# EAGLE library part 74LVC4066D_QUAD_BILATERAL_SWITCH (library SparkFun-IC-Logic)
Nexperia Quad Bilateral Switch The 74LVC4066 is a high-speed Si-gate CMOS device. The 74LVC4066 provides four single pole, single-throw analog switch functions. Each switch has two input/output terminals (nY and nZ) and an active HIGH enable input (nE). When nE is LOW, the analog switch is turned off. Schmitt-trigger action at the enable inputs makes the circuit tolerant of slower input rise and fall times across the entire VCC range from 1.65 V to 5.5 V. Datasheet
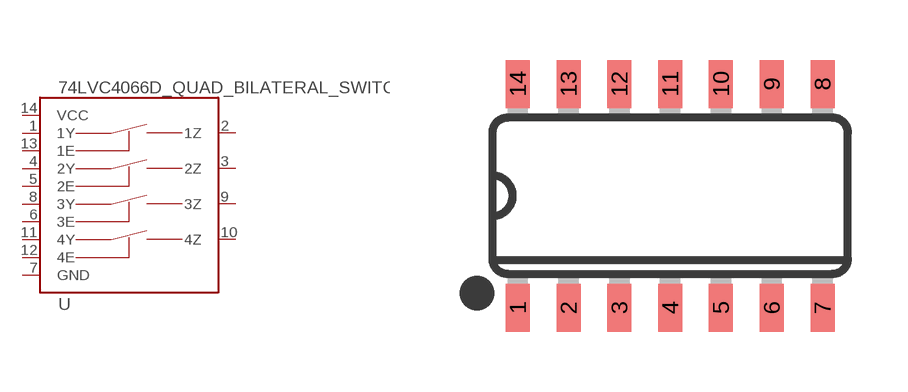
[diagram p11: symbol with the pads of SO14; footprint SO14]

Designator prefix U

## 74LVC4066D_QUAD_BILATERAL_SWITCH (PROD_ID: IC-13944)  [SO14]
1  1Y
2  1Z
3  2Z
4  2Y
5  2E
6  3E
7  GND
8  3Y
9  3Z
10  4Z
11  4Y
12  4E
13  1E
14  VCC

## Footprint SO14 (pad centres in mm)
smd 0.6 x 1.2: 1 -3.175,-2.8; 2 -1.905,-2.8; 3 -0.635,-2.8; 4 0.635,-2.8; 5 1.905,-2.8; 6 3.175,-2.8; 7 4.445,-2.8; 8 4.445,2.8; 9 3.175,2.8; 10 1.905,2.8; 11 0.635,2.8; 12 -0.635,2.8; 13 -1.905,2.8; 14 -3.175,2.8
